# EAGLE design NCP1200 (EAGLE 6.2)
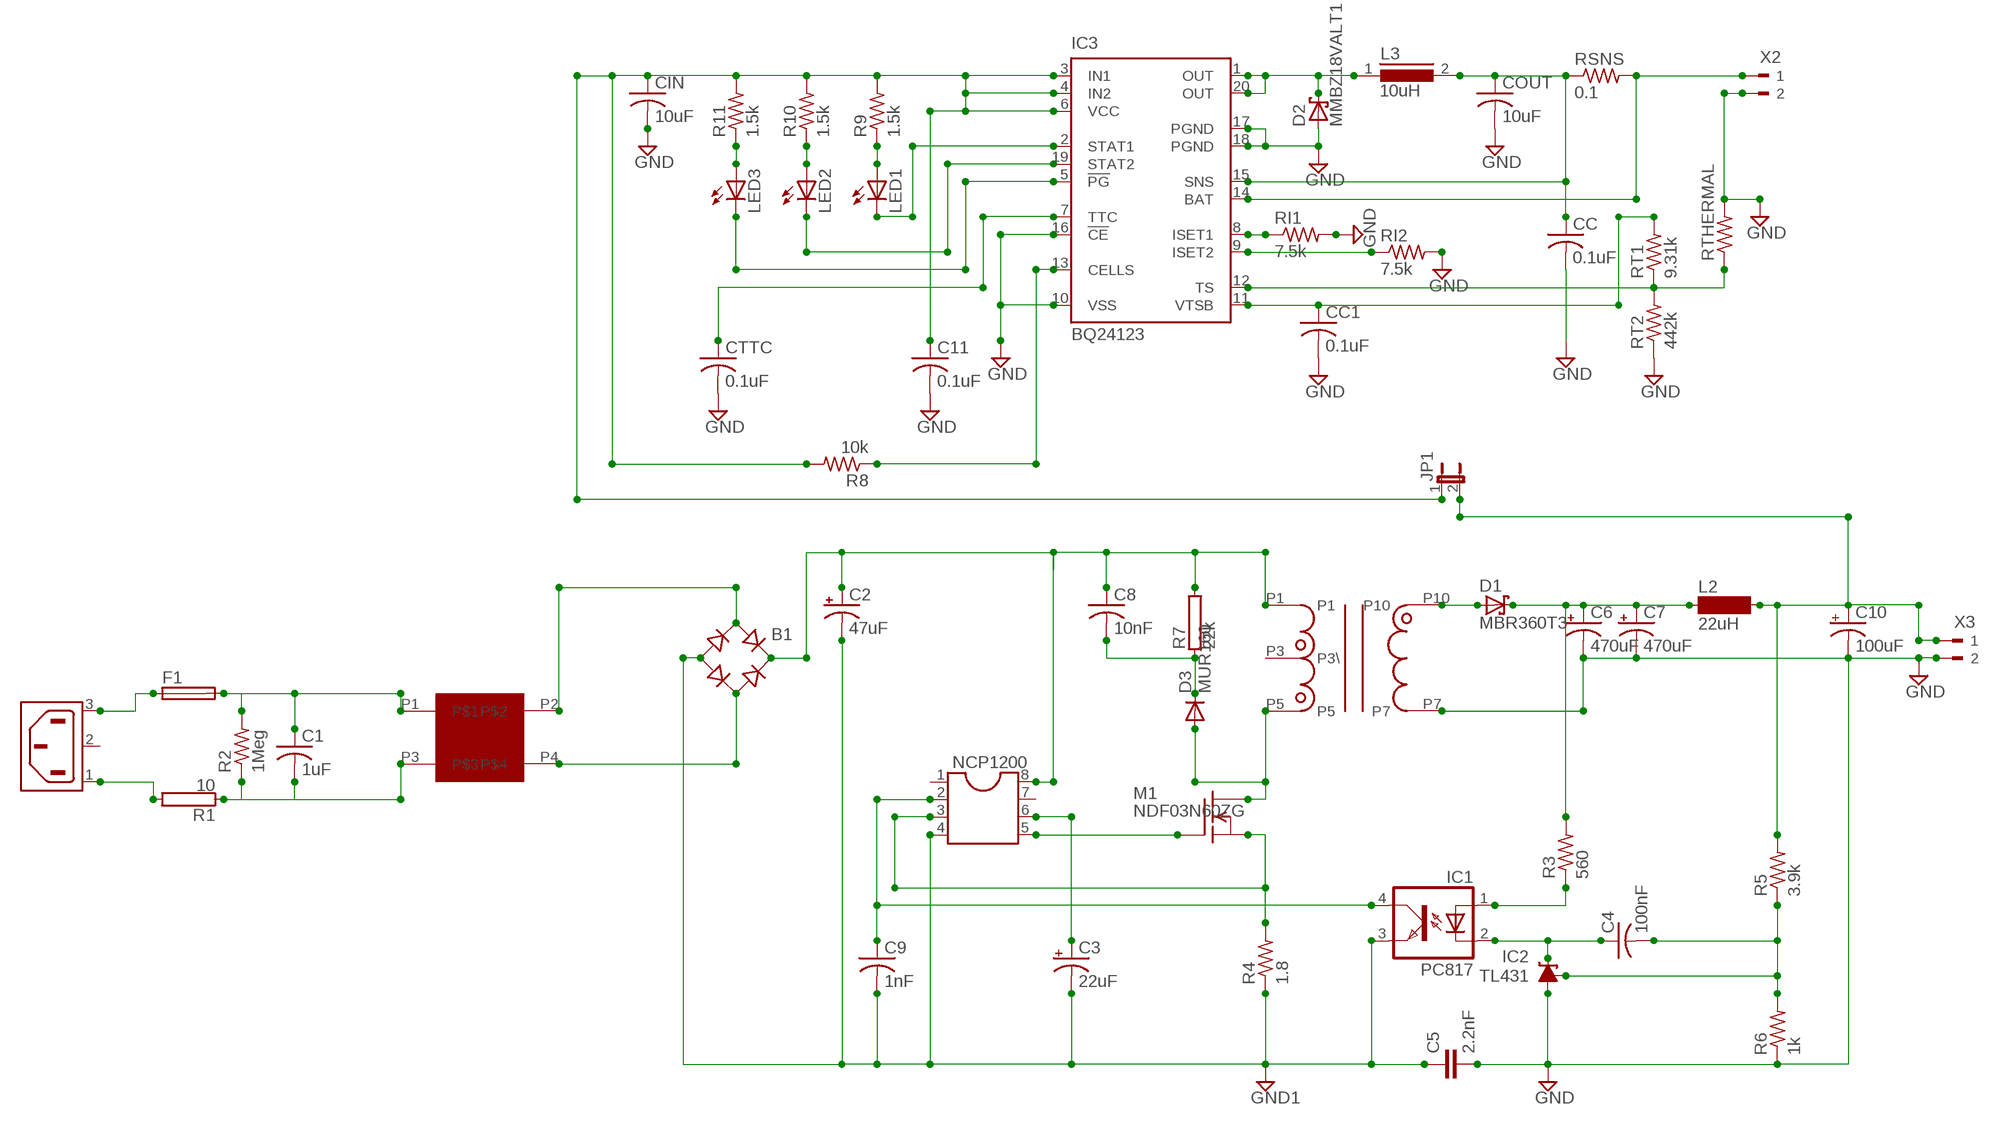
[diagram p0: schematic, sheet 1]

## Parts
B1  B-DIL  [B-DIL]
C1  1uF  C-US150-091X182  [C150-091X182]
C2  47uF  CPOL-USE10-22.5  [EB22,5D]
C3  22uF  CPOL-USE5-5  [E5-5]
C4  100nF  C-USC0805  [C0805]
C5  2.2nF  CYYC10B4  [YC10B4]
C6  470uF  CPOL-USE5-10.5  [E5-10,5]
C7  470uF  CPOL-USE5-10.5  [E5-10,5]
C8  10nF  C-US102-064X133  [C102-064X133]
C9  1nF  C-USC0805  [C0805]
C10  100uF  CPOL-USE2.5-6  [E2,5-6]
C11  0.1uF  C-USC0805  [C0805]
CC  0.1uF  C-USC0805  [C0805]
CC1  0.1uF  C-USC0805  [C0805]
CIN  10uF  C-USC0805  [C0805]
COUT  10uF  C-USC0805  [C0805]
CTTC  0.1uF  C-USC0805  [C0805]
D1  MBR360T3  MBRS130LT3  [SMB]
D2  MMBZ18VALT1  1N5908  [C4111-15]
D3  MUR160  BY203  [SGA-10]
F1  SH25  [SH25]
IC1  PC817  [DIL04]
IC2  TL431  LM4041BILP  [LP_O-PBCY-W3]
IC3  BQ24123  [QFN20_3,5X4,5]
JP1  JP1E  [JP1]
L2  22uH  SD8  [SD8]
L3  10uH  DR73  [DR73]
LED1  SFH482  [SFH482]
LED2  SFH482  [SFH482]
LED3  SFH482  [SFH482]
M1  NDF03N60ZG  BUZ20  [TO220]
NCP1200  DIL8  [DIL08]
R1  10  RKH206-8  [KH206-8]
R2  1Meg  R-US_R0805  [R0805]
R3  560  R-US_R0805  [R0805]
R4  1.8  R-US_R1206  [R1206]
R5  3.9k  R-US_R0805  [R0805]
R6  1k  R-US_R0805  [R0805]
R7  22k  RKH206-8  [KH206-8]
R8  10k  R-US_R0805  [R0805]
R9  1.5k  R-US_R0805  [R0805]
R10  1.5k  R-US_R0805  [R0805]
R11  1.5k  R-US_R0805  [R0805]
RI1  7.5k  R-US_R0805  [R0805]
RI2  7.5k  R-US_R0805  [R0805]
RSNS  0.1  R-US_R1206  [R1206]
RT1  9.31k  R-US_R0805  [R0805]
RT2  442k  R-US_R0805  [R0805]
RTHERMAL  R-US_R0805  [R0805]
U$1  RENCO1  [RENCO1]
U$2  L1CHO5  [L1CHO]
X1  6ESRM-P  [6ESRM-P]
X2  90-2  [90-2]
X3  90-2  [90-2]

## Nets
GND: C5.2 C6.- C7.- C10.- C11.2 CC1.2 CC.2 CIN.2 COUT.2 CTTC.2 D2.A IC2.3(A) IC3.10(VSS) IC3.16(!CE) IC3.17(PGND) IC3.18(PGND) R6.1 RI1.2 RI2.2 RT2.1 RTHERMAL.2 U$1.P7 X2.2 X3.2
N$1: D2.C IC3.1(OUT) IC3.20(OUT) L3.1
N$2: C1.2 R1.1 R2.1 U$2.P3
N$3: CC.1 COUT.1 IC3.15(SNS) L3.2 RSNS.1
N$4: B1.AC1 U$2.P2
N$5: B1.AC2 U$2.P4
N$6: IC3.8(ISET1) RI1.1
N$7: B1.+ C2.+ C8.1 NCP1200.8 R7.2 U$1.P1
N$8: C9.1 IC1.4(COL) NCP1200.2
N$9: M1.1(G) NCP1200.5
N$10: M1.3(S) NCP1200.3 R4.2
N$11: C3.+ NCP1200.6
N$12: C11.1 CIN.1 IC3.3(IN1) IC3.4(IN2) IC3.6(VCC) JP1.1 R8.2 R9.2 R10.2 R11.2
N$13: D1.A U$1.P10
N$14: C8.2 D3.C R7.1
N$15: D3.A M1.2(D) U$1.P5
N$16: C6.+ C7.+ D1.C L2.1 R3.2
N$17: IC1.1(A) R3.1
N$18: IC3.9(ISET2) RI2.1
N$19: C4.2 IC2.1(FB) R5.1 R6.2
N$20: C4.1 IC1.2(C) IC2.2(C)
N$21: IC3.12(TS) RT1.1 RT2.2 RTHERMAL.1
N$22: CC1.1 IC3.11(VTSB) RT1.2
N$23: LED3.A R11.1
N$24: LED2.A R10.1
N$25: LED1.A R9.1
N$26: IC3.2(STAT1) LED1.K(C)
N$27: IC3.19(STAT2) LED2.K(C)
N$28: IC3.5(!PG) LED3.K(C)
N$29: CTTC.1 IC3.7(TTC)
N$30: IC3.13(CELLS) R8.1
N$31: C1.1 F1.2 R2.2 U$2.P1
N$32: R1.2 X1.1(AC1)
N$33: IC3.14(BAT) RSNS.2 X2.1
N$34: F1.1 X1.3(AC2)
N$35: C10.+ JP1.2 L2.2 R5.2 X3.1
PE: B1.- C2.- C3.- C5.1 C9.2 IC1.3(EMIT) NCP1200.4 R4.1 ; supply symbol labelled GND1
Unconnected: IC3.EXP IC3.EXP@1 IC3.EXP@2 IC3.EXP@3 IC3.EXP@4 IC3.EXP@5 IC3.EXP@6 IC3.EXP@7 IC3.EXP@8 IC3.EXP@9 IC3.EXP@10 IC3.EXP@11 IC3.EXP@12 NCP1200.1 NCP1200.7 U$1.P3(P3\) X1.2(SH)

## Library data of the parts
B1 = rectifier:B-DIL: RECTIFIER
C1 C4 C8 C9 C11 CC CC1 CIN COUT CTTC = resistor:C-US: CAPACITOR, American symbol
C2 C3 C6 C7 C10 = resistor:CPOL-US: POLARIZED CAPACITOR, American symbol
C5 = resistor:CY: Y CAPACITOR
D1 = diode:MBRS130LT3: Schottky Power Rectifier
D2 = diode:1N5908: DIODE
D3 = diode:BY203: DIODE
F1 = fuse:SH25: FUSE HOLDER; MF: SCHURTER; MPN: 0031.8211; OC_FARNELL: 1162741; OC_NEWARK: 96B9380
IC1 = optocoupler:PC817: SHARP OPTO COUPLER; MPN: PC817X4J000F; OC_FARNELL: 9707727; OC_NEWARK: 97K7059
IC2 = texas:LM4041*I: PRECISION MICROPOWER SHUNT VOLTAGE REFERENCE Adjustable Output Source: http://focus.ti.com/lit/ds/slcs146e/slcs146e.pdf; OC_FARNELL: unknown; OC_NEWARK: unknown
IC3 = texas:BQ24123: SINGLE-CHIP SWITCHMODE, LI-ION AND LI-POLYMER CHARGE-MANAGEMENT IC WITH ENHANCED EMI PERFORMANCE(bqSWITCHER) Source: www.ti.com .. TI-bq24125.pdf; MPN: BQ24123RHLT; OC_FARNELL: 1407131; OC_NEWARK: 84K0851
JP1 = jumper:JP1E: JUMPER
L2 = inductor-neosid:SD8: INDUCTOR; OC_FARNELL: unknown; OC_NEWARK: unknown
L3 = inductors:DR73: High Power Density, High Efficiency, Shielded Inductors
LED1-LED3 = led:SFH482: IR LED
M1 = transistor-fet:BUZ20: N-Channel Enhancement MOSFET 100V; 12A; 0,2Ohm
NCP1200 = ic-package:DIL8: Dual In Line / Socket
R1 R7 = resistor-power:R: Power Resitor; OC_FARNELL: unknown; OC_NEWARK: unknown
R2-R6 R8-R11 RI1 RI2 RSNS RT1 RT2 RTHERMAL = resistor:R-US_: RESISTOR, American symbol
U$1 = renco:RENCO1
U$2 = l1choke:L1CHO5
X1 = con-tycoelectronics:6ESRM-P: AC Connector 120/250 VAC Source: http://catalog.tycoelectronics.com .. ENG_DS_1654001_1099_SR_0406.pdf; MF: TYCO ELECTRONICS; MPN: 6ESRM-P; OC_FARNELL: unknown; OC_NEWARK: 87F1821
X2 X3 = con-weidmueller-sl35:90-2: WEIDMUELLER CLAMP CONNECTOR; OC_FARNELL: unknown; OC_NEWARK: unknown

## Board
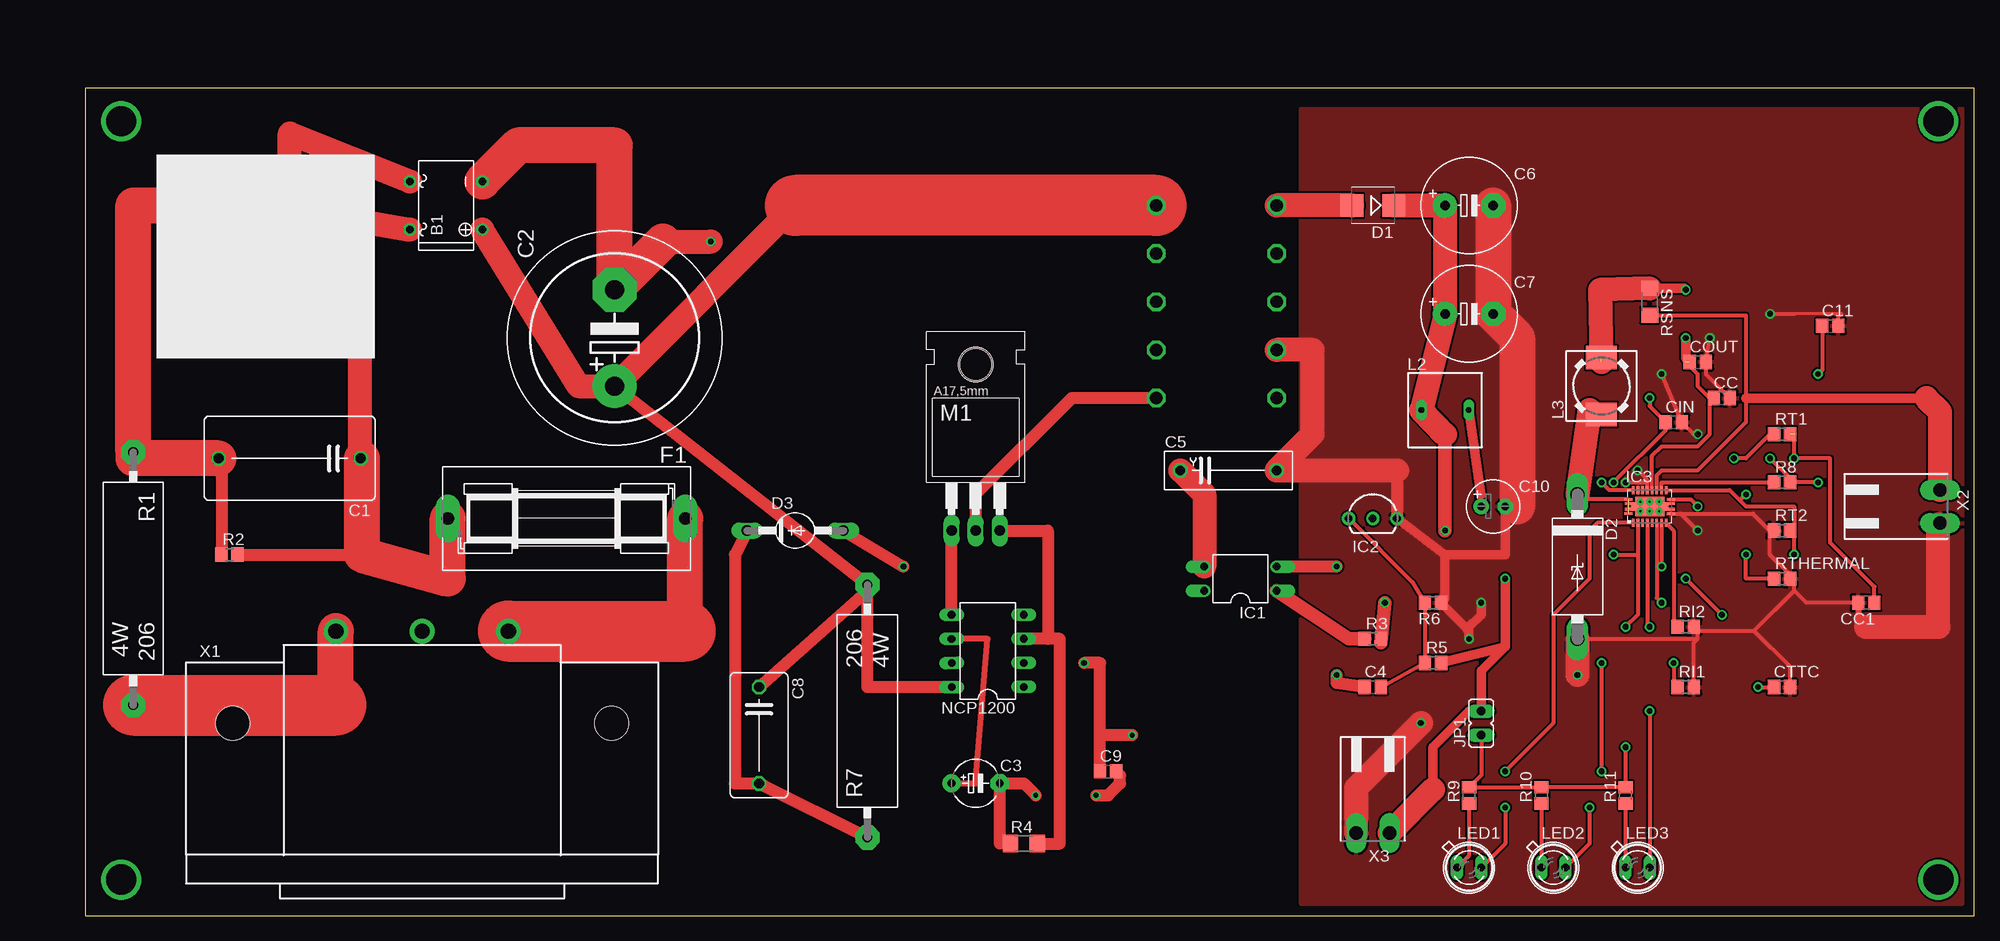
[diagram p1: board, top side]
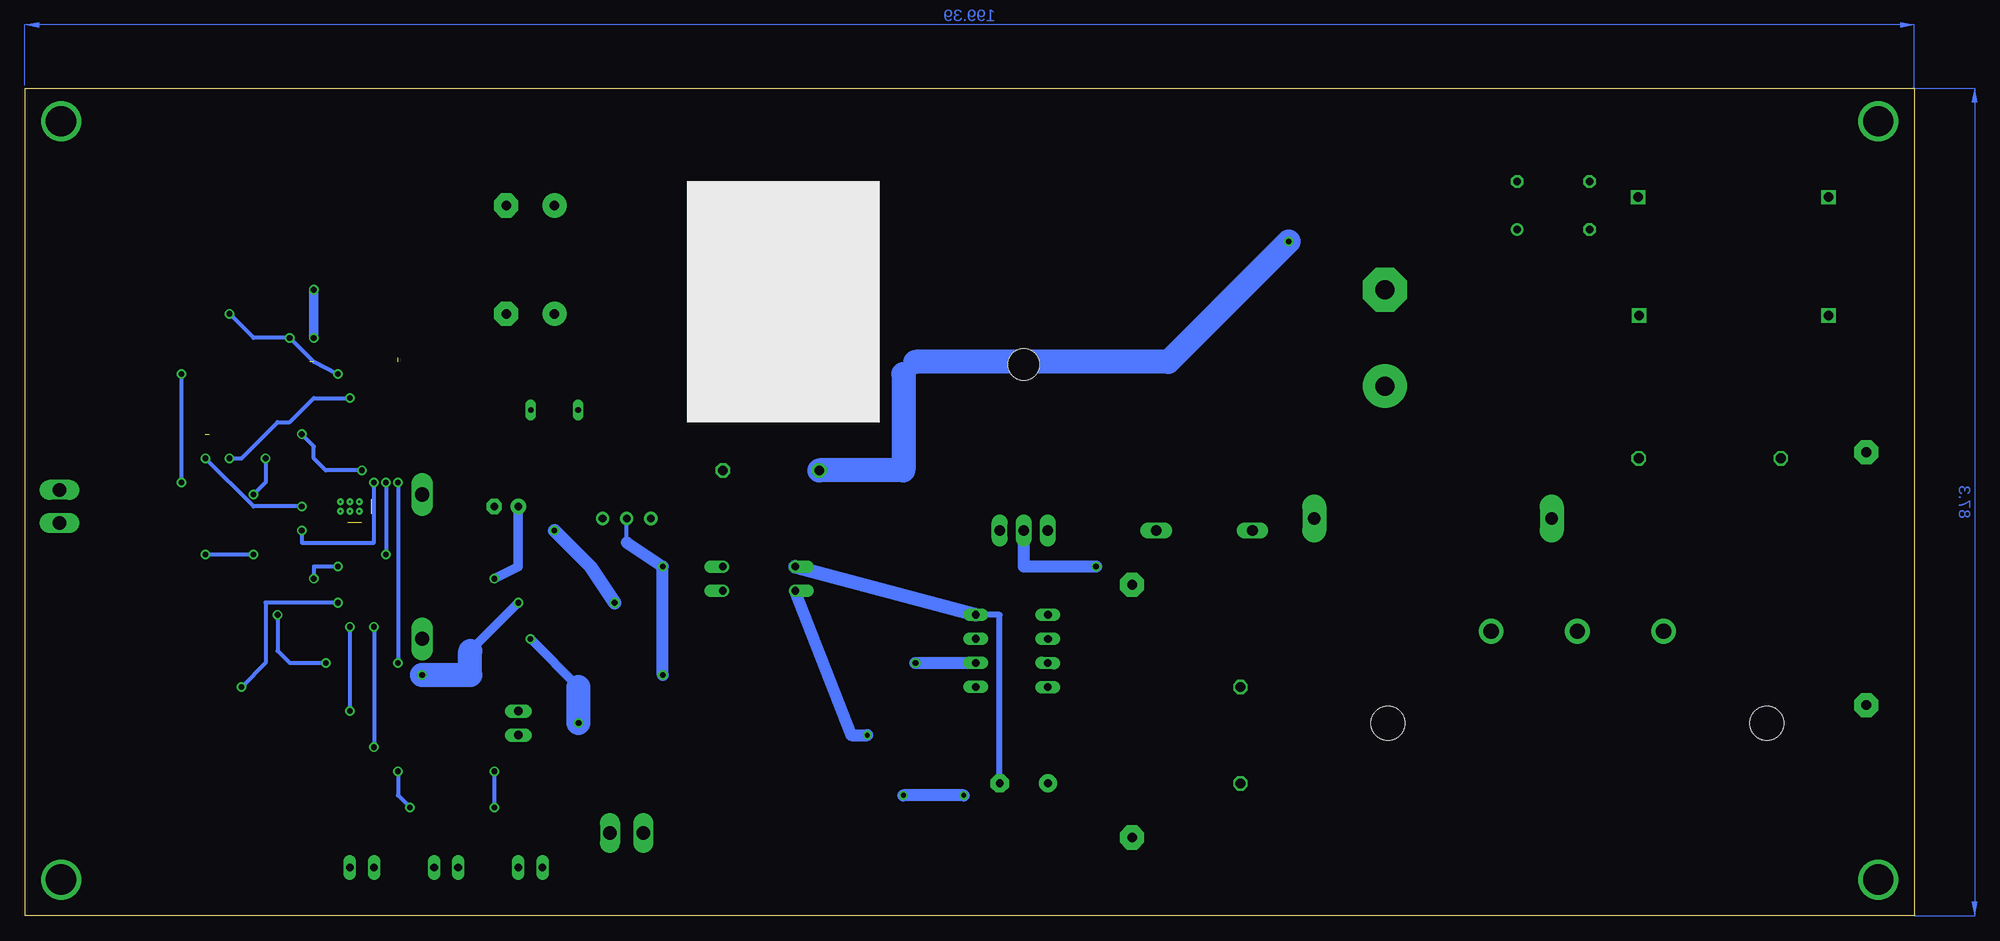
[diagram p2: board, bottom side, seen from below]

Size 199.37 x 87.3 mm. Coordinates in mm from the lower left corner, seen from the top.
Outline: 0,0 199.37,0 199.37,87.3 0,87.3 0,0
Copper layers (1*16): Top 0.035mm / dielectric 1.5mm / Bottom 0.035mm
Design rules: minimum track width 10mil, minimum drill 24mil, track to track 8mil, track to pad 8mil, pad to pad 8mil, via to via 8mil, smd to smd 8mil, copper to edge 40mil, drill to drill 8mil, minimum pad ring 10mil, minimum via ring 8mil, stop-mask expansion 4mil, vias tented up to drill 0mil, thermal gap 10mil

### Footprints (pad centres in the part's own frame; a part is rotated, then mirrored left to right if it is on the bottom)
B-DIL = drill 0.813: + -2.54,-3.81 | drill 0.813 octagon: - 2.54,-3.81; AC1 2.54,3.81; AC2 -2.54,3.81
C150-091X182 = drill 1.016 octagon: 1 -7.493,0; 2 7.493,0
EB22,5D = drill 2.007 pad 4.597: + -5.08,0 | drill 2.007 pad 4.597 octagon: - 5.08,0
E5-5 = drill 0.813 pad 1.905: + -2.54,0 | drill 0.813 pad 1.905 octagon: - 2.54,0
C0805 = smd 1.3 x 1.5: 1 -0.85,0; 2 0.85,0
YC10B4 = drill 1.016 octagon: 1 -5.08,0; 2 5.08,0
E5-10,5 = drill 1.016 pad 2.54: + -2.54,0 | drill 1.016 pad 2.54 octagon: - 2.54,0
C102-064X133 = drill 1.016 octagon: 1 -5.08,0; 2 5.08,0
E2,5-6 = drill 0.813 pad 1.6: + -1.27,0 | drill 0.813 pad 1.6 octagon: - 1.27,0
SMB = smd 2.4 x 2.4: A 2.2,0; C -2.2,0
C4111-15 = drill 1.499 long: A 7.62,0; C -7.62,0
SGA-10 = drill 1.118 long: A 5.08,0; C -5.08,0
SH25 = drill 1.321 pad 2.54 long: 1 -12.522,0; 2 12.522,0
DIL04 = drill 0.813 offset: 1 -1.27,-3.81; 2 1.27,-3.81; 3 1.27,3.81; 4 -1.27,3.81
LP_O-PBCY-W3 = drill 0.8 pad 1.4: 1 -2.54,0; 2 0,0; 3 2.54,0
QFN20_3,5X4,5 = smd 0.85 x 0.28: 1 -2.225,-0.75; 10 2.225,-0.75; 11 2.225,0.75; 20 -2.225,0.75 | smd 0.28 x 0.85: 2 -1.75,-1.725; 3 -1.25,-1.725; 4 -0.75,-1.725; 5 -0.25,-1.725; 6 0.25,-1.725; 7 0.75,-1.725; 8 1.25,-1.725; 9 1.75,-1.725; 12 1.75,1.725; 13 1.25,1.725; 14 0.75,1.725; 15 0.25,1.725; 16 -0.25,1.725; 17 -0.75,1.725; 18 -1.25,1.725; 19 -1.75,1.725 | smd 3.05 x 2.05: EXP 0,0 | drill 0.2 pad 0.3: EXP@1 -1,0.5; EXP@2 0,0.5; EXP@3 1,0.5; EXP@4 -1,-0.5; EXP@5 0,-0.5; EXP@6 1,-0.5 | smd 1.125 x 0.28: EXP@7 -2.075,0.3; EXP@8 -2.075,-0.3; EXP@9 2.075,0.3; EXP@10 2.075,-0.3 | smd 0.45 x 0.4: EXP@11 -1.75,0; EXP@12 1.75,0
JP1 = drill 0.914 long: 1 0,-1.27; 2 0,1.27
SD8 = drill 0.6 long: 1 -2.5,0; 2 2.5,0
DR73 = smd 2.5 x 3.25: 1 -3,0; 2 3,0
SFH482 = drill 0.813 long: A -1.27,0; K 1.27,0
TO220 = drill 1.118 long: 1 -2.54,-6.35; 2 0,-6.35; 3 2.54,-6.35 | hole 3.302: 0,11.176
DIL08 = drill 0.813 long: 1 -3.81,-3.81; 2 -1.27,-3.81; 3 1.27,-3.81; 4 3.81,-3.81; 5 3.81,3.81; 6 1.27,3.81; 7 -1.27,3.81; 8 -3.81,3.81
KH206-8 = drill 1.016 pad 2.54 octagon: 1 -13.335,0; 2 13.335,0
R0805 = smd 1.3 x 1.5: 1 -0.85,0; 2 0.85,0
R1206 = smd 1.6 x 1.803: 1 -1.422,0; 2 1.422,0
RENCO1 = drill 1.3 octagon: P1 -10.16,5.08; P2 -5.08,5.08; P3 0,5.08; P4 5.08,5.08; P5 10.16,5.08; P6 10.16,-7.62; P7 5.08,-7.62; P8 0,-7.62; P9 -5.08,-7.62; P10 -10.16,-7.62
L1CHO = drill 1 square: P1 -10,4; P2 10,4; P3 10,-8.5; P4 -10.1,-8.5
6ESRM-P = drill 1.6 pad 2.6: 1 -9.1,9.7; 2 0,9.7; 3 9.1,9.7 | hole 3.6: -20,0; 20,0
90-2 = drill 1.422 long: 1 -1.75,5.25; 2 1.75,5.25

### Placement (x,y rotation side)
B1  38.1,74.93 90 top
C1  21.59,48.26 180 top
C2  55.88,60.96 90 top
C3  93.98,13.97 0 top
C4  135.89,24.13 0 top
C5  120.65,46.99 0 top
C6  146.05,74.93 0 top
C7  146.05,63.5 0 top
C8  71.12,19.05 270 top
C9  107.95,15.24 0 top
C10  148.59,43.18 0 top
C11  184.15,62.23 0 top
CC  172.72,54.61 0 top
CC1  187.96,33.02 180 top
CIN  167.64,52.07 0 top
COUT  170.18,58.42 0 top
CTTC  179.07,24.13 0 top
D1  135.89,74.93 180 top
D2  157.48,36.83 270 top
D3  74.93,40.64 0 top
F1  50.8,41.91 180 top
IC1  121.92,35.56 90 top
IC2  135.89,41.91 0 top
IC3  165.1,43.18 0 top
JP1  147.32,20.32 0 top
L2  143.51,53.34 0 top
L3  160.02,55.88 90 top
LED1  146.05,5.08 0 top
LED2  154.94,5.08 0 top
LED3  163.83,5.08 0 top
M1  93.98,46.99 0 top
NCP1200  95.25,27.94 90.1 top
R1  5.08,35.56 270 top
R2  15.24,38.1 0 top
R3  135.89,29.21 0 top
R4  99.06,7.62 0 top
R5  142.24,26.67 0 top
R6  142.24,33.02 180 top
R7  82.55,21.59 90 top
R8  179.07,45.72 0 top
R9  146.05,12.7 90 top
R10  153.67,12.7 90 top
R11  162.56,12.7 90 top
RI1  168.91,24.13 0 top
RI2  168.91,30.48 0 top
RSNS  165.1,64.77 270 top
RT1  179.07,50.8 0 top
RT2  179.07,40.64 0 top
RTHERMAL  179.07,35.56 0 top
U$1  118.11,64.77 270 bottom
U$2  19.05,67.31 180 top
X1  35.56,20.32 0 top
X2  190.5,43.18 270 top
X3  135.89,13.97 180 top

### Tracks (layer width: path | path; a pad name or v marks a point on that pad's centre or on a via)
GND  (via drill 0.6)
  Top 0.305: C11.2 185,63.08 185.42,63.5 180.34,63.5
  Top 0.406: v171.45,60.96 COUT.2 171.03,57.15 CC.2 | v177.8,63.5 180.34,63.5 | v166.37,57.15 CIN.2 169.76,50.8 v170.18,50.8 | 177.8,40.64 176.01,42.43 IC3.10 168.39,42.43 v170.18,40.64 | IC3.16 164.85,45.72 | 164.85,45.72 164.85,45.97 v163.83,46.99 | D2.A 170.18,29.21 | 170.18,29.21 170.18,30.06 | 170.18,30.06 RI2.2 | RI1.2 169.76,28.79 170.18,29.21 | 170.18,30.06 176.11,30.06 | 176.11,30.06 180.34,34.29 | 180.34,34.29 180.34,35.56 | CTTC.2 179.92,26.25 176.11,30.06 | 195.75,40.81 X2.2 195.58,41.26 | 180.34,34.29 181.61,33.02 CC1.2 187.11,32.84 | 187.11,31.33 187.96,30.48 | RTHERMAL.2 179.92,35.98 177.8,38.1 177.8,40.22 RT2.1 | v162.56,45.72 164.85,45.72 | 151.13,43.18 C10.- | R6.1 143.51,33.44 | 146.05,30.06 145.84,30.27
  Top 0.61: CC1.2 187.11,31.33
  Top 1.016: IC2.3 143.51,38.1 | 143.51,38.1 149.86,38.1 C10.- | 143.51,33.44 143.51,38.1 | v146.05,29.21 146.05,30.06 | R6.1 145.84,30.27 147.32,31.75 v147.32,33.02
  Top 1.27: 138.43,46.99 IC2.3
  Top 2.54: 187.96,30.48 195.58,30.48 195.58,41.26 | U$1.P7 129.54,59.69 129.54,50.8 C5.2 138.43,46.99 | X3.2 134.14,13.49 v140.97,20.32 | D2.A v157.48,25.4
  Top 3.81: C6.- C7.- 151.13,60.96 151.13,43.18
  Bottom 0.406: v177.8,63.5 175.26,60.96 v171.45,60.96 168.91,58.42 v166.37,57.15 | v163.83,46.99 167.64,46.99 168.91,48.26 168.91,49.53 v170.18,50.8 | v170.18,40.64 170.18,39.37 162.56,39.37 v162.56,45.72
  Bottom 1.016: 140.97,24.13 v146.05,29.21 | 152.4,27.94 v147.32,33.02
  Bottom 2.54: v140.97,20.32 140.97,24.13 | v157.48,25.4 152.4,25.4 152.4,27.94
  pour Top: 198.12,1.27 198.12,85.09 128.27,85.09 128.27,1.27
N$1  (1 unrouted)
  Top 0.406: L3.1 158.75,53.34 | IC3.20 158,43.93 D2.C
  Top 2.54: 158.75,53.34 D2.C
N$2
  Top 0.406: C1.2 14.39,48.26 | 5.08,48.26 R1.1 | 9.05,74.93 U$2.P3
  Top 1.27: 14.39,48.26 R2.1
  Top 3.81: C1.2 5.08,48.26 | R1.1 5.08,74.93 9.05,74.93
N$3  (via drill 0.6)  (2 unrouted)
  Top 0.406: IC3.15 165.35,48.51 166.37,49.53 170.18,49.53 171.45,50.8 171.45,54.19 CC.1 171.45,54.61 170.18,55.88 170.18,57.15 168.91,58.42 | 168.76,66.19 v168.91,66.04 | 168.91,58.84 COUT.1
  Top 1.016: RSNS.1 168.76,66.19 | v168.91,60.96 168.91,58.84
  Top 2.54: RSNS.1 159.87,66.04 160.02,58.42
  Bottom 1.016: v168.91,66.04 v168.91,60.96
N$4
  Top 2.54: U$2.P2 21.59,63.31 21.59,82.55 B1.AC1
N$5
  Top 2.54: U$2.P4 29.21,73.27 B1.AC2
N$6  (via drill 0.6)
  Top 0.406: IC3.8 166.35,36.85 v166.37,36.83 | v168.91,35.56 v172.72,31.75 | v167.64,26.67 167.64,24.55 RI1.1
  Bottom 0.406: v166.37,36.83 168.91,36.83 v168.91,35.56 | v172.72,31.75 172.72,27.94 171.45,26.67 v167.64,26.67
N$7
  Top 0.406: 82.55,34.29 R7.2
  Top 1.27: C8.1 82.55,34.29 82.55,24.12 NCP1200.8 | C2.+ R7.2
  Top 2.54: B1.+ 52.07,55.88 C2.+ 74.93,74.93
  Top 6.452: U$1.P1 74.93,74.93
N$8  (via drill 0.5, 0.6)
  Top 1.27: C9.1 107.1,19.05 | 107.1,19.05 107.1,26.67 v105.41,26.67 | v110.49,19.05 107.1,19.05
  Bottom 0.406: v105.41,26.67 v105.41,26.68
  Bottom 1.27: v105.41,26.68 NCP1200.2 | IC1.4 112.18,19.05 v110.49,19.05
N$9
  Top 0.406: NCP1200.5
  Top 1.27: NCP1200.5 M1.1
N$10
  Top 0.406: NCP1200.3
  Top 1.27: R4.2 102.87,7.62 102.87,29.21 101.6,29.21 | 101.6,29.21 NCP1200.3 | M1.3 101.6,40.64 101.6,29.21
N$11
  Top 0.406: NCP1200.6
  Top 0.61: C3.+ 93.98,13.97 95.25,29.21 NCP1200.6
N$12  (via drill 0.6)  (2 unrouted)
  Top 0.406: v161.29,45.72 166.79,51.22 CIN.1 165.1,53.76 v165.1,54.61 | v161.29,38.1 163.83,38.1 | IC3.3 163.83,41.44 163.83,38.1 | C11.1 183.3,57.57 v182.88,57.15 | v182.88,45.72 R8.2 179.92,46.14 v177.8,48.26 | 163.83,38.1 163.83,31.75 v162.56,30.48 | v162.56,17.78 R11.2 R10.2 R9.2 147.32,14.82 JP1.1
  Bottom 0.406: v161.29,45.72 v161.29,38.1 | v182.88,57.15 v182.88,45.72 | v177.8,48.26 176.53,48.26 172.72,52.07 171.45,52.07 168.91,54.61 v165.1,54.61 | v162.56,30.48 v162.56,17.78
N$13
  Top 2.54: D1.A U$1.P10
N$14
  Top 1.27: D3.C 68.58,38.1 68.58,13.97 C8.2 R7.1
N$15  (via drill 0.6)
  Top 1.27: D3.A v86.36,36.83 | U$1.P5 104.14,54.61 93.98,44.45 M1.2
  Bottom 1.27: v86.36,36.83 93.98,36.83 M1.2
N$16  (via drill 0.6)
  Top 0.406: C7.+ 143.55,63.46 | 136.74,28.79 R3.2
  Top 1.422: 143.51,50.76 v143.51,40.64 | v137.16,33.02 136.74,28.79
  Top 2.54: D1.C C6.+ C7.+ | 143.55,63.46 L2.1 143.51,50.76
  Bottom 1.422: v143.51,40.64 139.7,36.83 v137.16,33.02
N$17
  Top 1.422: IC1.1 133.35,29.21 R3.1
N$18
  Top 0.406: IC3.9 166.85,41.43 167.64,40.64 167.64,30.9 RI2.1
N$19
  Top 0.406: IC2.1 140.12,35.14 R6.2 R5.1 C4.2
N$20  (via drill 0.6)
  Top 1.27: C4.1 132.08,24.55 v132.08,25.4 | v132.08,36.83 IC1.2
  Bottom 0.406: 135.89,39.37 IC2.2
  Bottom 1.27: v132.08,25.4 v132.08,36.83 135.89,39.37
N$21  (via drill 0.6)
  Top 0.406: IC3.12 173.53,44.91 174.62,43.81 | 174.62,43.81 175.26,43.18 180.34,43.18 180.34,41.06 RT2.2 180.34,40.64 v180.34,38.1 | RT1.1 177.8,50.8 175.26,48.26 v173.99,48.26 | v175.26,44.45 174.62,43.81 | RTHERMAL.1 175.26,35.56 v175.26,38.1
  Bottom 0.406: v173.99,48.26 173.99,45.72 v175.26,44.45 | v175.26,38.1 v180.34,38.1
N$22  (via drill 0.6)  (1 unrouted)
  Top 0.406: IC3.11 169.43,43.93 v170.18,43.18 | 180.34,50.8 v180.34,48.26 184.15,48.26 184.15,39.37 188.81,34.71 CC1.1
  Bottom 0.406: v170.18,43.18 175.26,43.18 v180.34,48.26
N$23
  Top 0.406: R11.1 LED3.A
N$24
  Top 0.406: R10.1 LED2.A
N$25
  Top 0.406: R9.1 146.05,6.35 LED1.A
N$26  (via drill 0.6)
  Top 0.406: IC3.2 159.56,41.45 158.75,40.64 158.75,35.56 154.94,31.75 154.94,20.32 v149.86,15.24 | v149.86,11.43 149.86,7.62 LED1.K
  Bottom 0.406: v149.86,15.24 v149.86,11.43
N$27  (via drill 0.6)
  Top 0.406: IC3.19 160.84,44.91 v160.02,45.72 | v160.02,26.67 v160.02,15.24 | v158.75,11.43 158.75,7.62 LED2.K
  Bottom 0.406: v160.02,45.72 v160.02,26.67 | v160.02,15.24 160.02,12.7 v158.75,11.43
N$28  (via drill 0.6)
  Top 0.406: IC3.5 164.85,30.73 v165.1,30.48 | v165.1,21.59 LED3.K
  Bottom 0.406: v165.1,30.48 v165.1,21.59
N$29  (via drill 0.6)
  Top 0.406: IC3.7 165.85,33.54 v166.37,33.02 | v176.53,24.13 CTTC.1
  Bottom 0.406: v166.37,33.02 173.99,33.02 173.99,26.67 v176.53,24.13
N$30
  Top 0.406: IC3.13 166.35,45.7 166.37,45.72 R8.1
N$31
  Top 0.406: 29.21,48.26 C1.1 29.05,48.26
  Top 1.27: R2.2 29.21,38.1
  Top 2.54: 29.05,48.26 U$2.P1
  Top 3.81: F1.2 38.28,35.56 29.21,38.1 29.21,48.26
N$32
  Top 3.81: 26.46,22.23 X1.1
  Top 6.452: R1.2 26.46,22.23
N$33
  Top 0.406: RSNS.2 175.26,63.35 175.26,54.61 175.26,52.07 170.18,46.99 166.37,46.99 165.85,46.47 IC3.14
  Top 1.016: 194.31,54.61 175.26,54.61
  Top 2.54: X2.1 195.75,53.17 194.31,54.61
N$34
  Top 3.81: 63.32,30.02 F1.1
  Top 6.452: X1.3 63.32,30.02
N$35  (via drill 0.6)
  Top 0.406: C10.+ 147.28,44.41
  Top 1.016: 147.28,44.41 L2.2 | R5.2 149.86,28.36 | 149.86,28.36 v149.86,35.56 | 149.86,28.36 147.32,25.82 JP1.2 146.05,21.59 142.24,17.78 142.24,13.32
  Top 2.54: 142.24,13.32 X3.1
  Bottom 1.016: v149.86,35.56 147.32,36.83 C10.+
N$37  (via drill 3.2)
  other vias: 3.81,83.82
N$38  (via drill 3.2)
  other vias: 195.58,83.82
N$39  (via drill 3.2)
  other vias: 195.58,3.81
N$40  (via drill 3.2)
  other vias: 3.81,3.81
PE  (via drill 0.5, 0.6)
  Top 0.305: 109.22,14.82 C9.2
  Top 0.406: R4.1 96.52,7.62
  Top 1.27: 96.52,7.62 C3.- 99.06,13.97 v100.33,12.7 | v106.68,12.7 107.95,12.7 109.22,13.97 109.22,14.82
  Top 2.54: C5.1 118.11,44.45 IC1.3 | 60.96,71.12 v66.04,71.12
  Top 3.81: 60.96,71.12 C2.- 55.88,81.28 45.72,81.28 B1.-
  Bottom 0.406: 105.41,58.42 106.68,57.15
  Bottom 0.61: C3.- 96.52,31.75 NCP1200.4
  Bottom 1.27: v100.33,12.7 v106.68,12.7
  Bottom 1.422: NCP1200.4 IC1.3
  Bottom 2.54: v66.04,71.12 78.74,58.42 105.41,58.42 | 106.68,57.15 106.68,46.99 C5.1
(copper drawn outside any net)
  shapes: Bottom area x2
